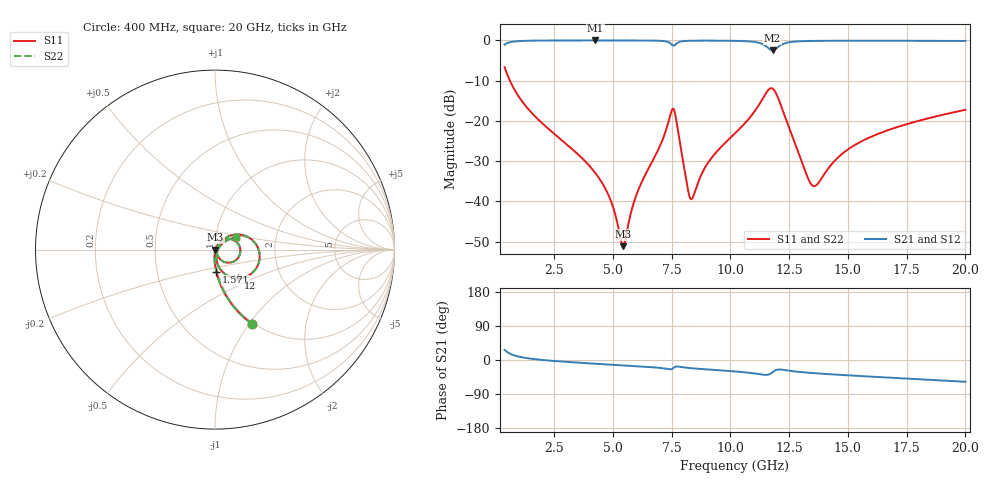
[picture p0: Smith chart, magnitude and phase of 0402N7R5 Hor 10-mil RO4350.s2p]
# GHz S MA R 50
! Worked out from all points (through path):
!   1960 points, 400 MHz to 20 GHz, reference 50 ohm
!   highest |S21| = -0.02 dB at 4.252 GHz (marker M1); lowest = -2.5 dB at 11.8 GHz (marker M2)
!   group delay of S21, straight-line fit = 8.76 ps
!   lowest |S11| = -51.1 dB at 5.443 GHz (marker M3), VSWR 1.01, Z = 50.3 - j0.0718 ohm
!   |S11| at or under -10 dB: 624.8 MHz to end of sweep
!   |S22| runs from -51.1 to -6.7 dB; largest |S21 - S12| = 0
!   S11 on the Smith chart (normalised r, x): 400 MHz: 0.98, -1.04; 1.571 GHz: 0.98, -0.25; 12 GHz: 1.22, -0.41; 20 GHz: 1.26, +0.17
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0.4  0.4641 -63.3  0.8854 26.6  0.8854 26.6  0.4641 -63.3
0.8002042  0.2503 -77.4  0.9675 12.4  0.9675 12.4  0.2503 -77.4
1.570597  0.1241 -86.5  0.9911 3.0  0.9911 3.0  0.1241 -86.5
3.671669  0.0349 -94.4  0.9973 -7.6  0.9973 -7.6  0.0349 -94.4
4.251965  0.02264 -94.4  0.9974 -9.8  0.9974 -9.8  0.02264 -94.4
4.892292  0.01062 -88.9  0.9973 -12.1  0.9973 -12.1  0.01062 -88.9
5.442573  0.002774 -14.9  0.997 -14.1  0.997 -14.1  0.002774 -14.9
6.022869  0.01238 57.6  0.9962 -16.3  0.9962 -16.3  0.01238 57.6
6.943338  0.04437 57.7  0.9896 -20.5  0.9896 -20.5  0.04437 57.7
7.59367  0.1392 -15.4  0.861 -20.3  0.861 -20.3  0.1392 -15.4
8.193977  0.01416 -44.4  0.9867 -20.9  0.9867 -20.9  0.01416 -44.4
8.354058  0.01064 -2.6  0.9896 -21.8  0.9896 -21.8  0.01064 -2.6
9.054416  0.03021 51.7  0.9923 -25.0  0.9923 -25.0  0.03021 51.7
10.205  0.07004 50.8  0.9862 -30.2  0.9862 -30.2  0.07004 50.8
11.34558  0.1817 25.5  0.9064 -38.5  0.9064 -38.5  0.1817 25.5
11.79581  0.2522 -24.4  0.749 -32.1  0.749 -32.1  0.2522 -24.4
11.99592  0.2041 -51.6  0.8121 -25.5  0.8121 -25.5  0.2041 -51.6
12.42614  0.09402 -78.2  0.9372 -27.6  0.9372 -27.6  0.09402 -78.2
13.46667  0.01596 -34.5  0.9835 -34.3  0.9835 -34.3  0.01596 -34.5
14.97744  0.0436 38.0  0.9897 -40.4  0.9897 -40.4  0.0436 38.0
16.73834  0.07716 38.2  0.9892 -46.5  0.9892 -46.5  0.07716 38.2
20  0.1373 29.7  0.9829 -57.4  0.9829 -57.4  0.1373 29.7
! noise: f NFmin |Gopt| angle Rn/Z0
0.4  0.001012  0.7413  2.408  0.0007842
2.571  0.005148  0.6827  6.988  0.003132
4.752  0.008745  0.6609  12.43  0.004876
6.933  0.02027  0.7738  17.89  0.01787
9.104  0.02045  0.7177  23.38  0.01375
11.29  0.07218  0.8922  28.86  0.1368
13.47  0.03724  0.7701  34.27  0.03019
15.64  0.0282  0.6725  39.22  0.01479
17.82  0.02804  0.639  44.01  0.0127
20  0.02945  0.6251  48.65  0.01234
